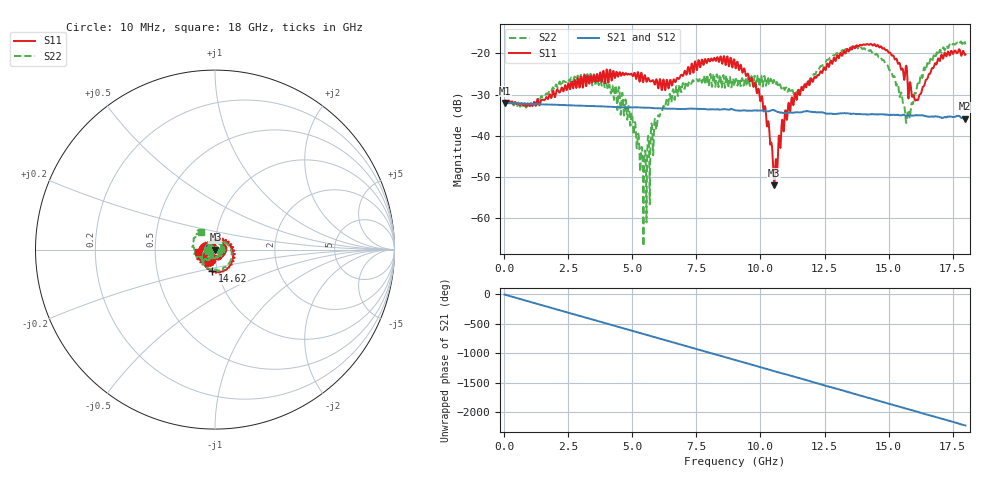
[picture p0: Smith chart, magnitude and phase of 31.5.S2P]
!Agilent Technologies,E5071C,MY46316741,A.11.02
!Date: Fri May 06 15:20:39 2022
!Data & Calibration Information:
!Freq	S11:SOLT2(ON)	S21:SOLT2(ON)	S12:SOLT2(ON)	S22:SOLT2(ON)
!PortZ  Port1:50+j0  Port2:50+j0
!Above PortZ is port z conversion or system Z0 setting when saving the data.
!When reading, reference impedance value at option line is always used.
# Hz S dB R 50
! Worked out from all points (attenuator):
!   1800 points, 10 MHz to 18 GHz, reference 50 ohm
!   highest |S21| = -32.01 dB at 10 MHz (marker M1); lowest = -35.8 dB at 17.98 GHz (marker M2)
!   lowest |S11| = -52.0 dB at 10.54 GHz (marker M3), VSWR 1.01, Z = 50.2 - j0.12 ohm
!   |S11| at or under -10 dB: start of sweep to end of sweep
!   |S22| runs from -66.8 to -16.8 dB; largest |S21 - S12| = 0.0015
!   S11 on the Smith chart (normalised r, x): 10 MHz: 0.95, +0.00; 14.62 GHz: 0.94, -0.23; 18 GHz: 0.82, -0.02
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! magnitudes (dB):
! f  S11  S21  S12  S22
! 10 MHz  -31.5  -32.0  -32.0  -31.7
! 1.03 GHz  -32.1  -32.2  -32.3  -32.3
! 3.01 GHz  -25.6  -32.7  -32.7  -25.5
! 4.67 GHz  -25.2  -33.1  -33.1  -35.1
! 5.17 GHz  -25.6  -33.1  -33.1  -43.0
! 5.48 GHz  -25.3  -33.2  -33.2  -44.0
! 6.01 GHz  -28.5  -33.3  -33.3  -35.0
! 7.16 GHz  -23.7  -33.4  -33.4  -27.9
! 9.01 GHz  -22.9  -33.8  -33.8  -27.2
! 9.99 GHz  -31.5  -33.9  -33.9  -26.7
! 10.54 GHz  -52.0  -33.8  -33.9  -26.7
! 11.04 GHz  -35.8  -34.3  -34.4  -29.1
! 12.01 GHz  -26.5  -34.2  -34.3  -26.1
! 13.26 GHz  -19.4  -34.5  -34.5  -19.3
! 14.62 GHz  -18.4  -34.8  -34.8  -20.9
! 15.01 GHz  -19.8  -34.9  -34.9  -23.7
! 15.75 GHz  -28.0  -35.1  -35.0  -33.9
! 16.1 GHz  -31.2  -35.0  -35.1  -28.5
! 16.58 GHz  -25.0  -35.3  -35.4  -22.9
! 17.13 GHz  -21.3  -35.6  -35.7  -18.6
! 17.98 GHz  -20.4  -35.8  -36.0  -17.4
! 18 GHz  -20.3  -35.8  -36.0  -17.8
